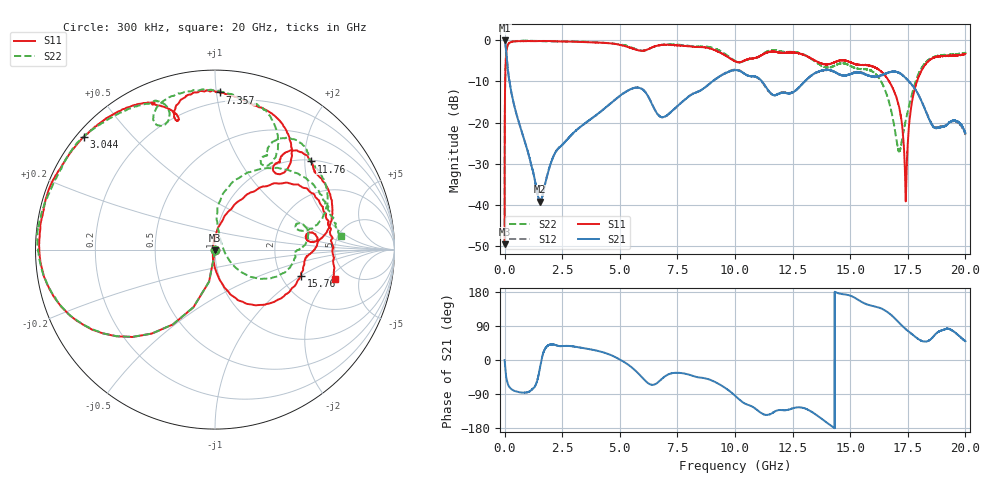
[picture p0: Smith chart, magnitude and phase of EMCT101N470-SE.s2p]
!EMCT101N470
!Johanson Technology Inc.
!www.johansontechnology.com
!Test Board Conditions:
!Substrate Type  RO4350B
!Substrate Thickness  10 mil
!Substrate Dk  3.66
!TL Type: GCPW
!TL Trace Width  22 mil
!TL Gap  14 mil
!PART MODE SINGLE ENDED (AKA BYPASS)
!DUT TOPOLOGY	SERIES-SHUNT
# MHz S  dB  R 50
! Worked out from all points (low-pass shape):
!   20001 points, 300 kHz to 20 GHz, reference 50 ohm
!   highest |S21| = -0.01 dB at 1.3 MHz (marker M1); lowest = -39.2 dB at 1.536 GHz (marker M2)
!   |S21| within 3 dB of the highest: start of sweep to 70.19 MHz
!   lowest |S11| = -49.6 dB at 300 kHz (marker M3), VSWR 1.01, Z = 50.2 - j0.292 ohm
!   |S11| at or under -10 dB: start of sweep to 23.99 MHz; 16.69105 GHz to 16.69105 GHz (0 Hz wide, 0 % of centre); 16.69 GHz to 17.9 GHz (1.208 GHz wide, 6.99 % of centre)
!   |S22| runs from -50.1 to 0.0 dB; largest |S21 - S12| = 0.0096
!   S11 on the Smith chart (normalised r, x): 300 kHz: 1.00, -0.01; 3.044 GHz: 0.02, +0.37; 7.357 GHz: 0.14, +1.02; 11.76 GHz: 1.03, +2.15; 15.76 GHz: 2.55, -1.00; 20 GHz: 3.79, -2.40
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0.3  -49.62 -61.7  -0.02 -0.4  -0.01 -0.3  -50.10 -65.6
1.3  -35.02 -87.8  -0.01 -1.1  -0.01 -1.1  -35.01 -87.5
101.298  -1.84 -146.2  -4.90 -55.2  -4.87 -55.2  -1.87 -146.0
157.298  -0.92 -157.6  -7.85 -65.9  -7.81 -66.0  -0.93 -157.1
1536.277  -0.14 164.4  -39.24 -20.0  -39.09 -19.3  -0.15 164.5
2172.267  -0.20 154.2  -27.64 40.2  -27.57 40.1  -0.27 155.7
3044.254  -0.33 139.3  -22.22 35.2  -22.23 34.9  -0.24 144.1
3334.25  -0.38 135.1  -20.84 32.2  -20.86 32.1  -0.27 140.6
5687.215  -2.22 105.6  -11.51 -28.5  -11.47 -28.2  -2.09 108.8
6667.2  -1.23 100.7  -18.16 -58.5  -18.11 -58.9  -1.21 110.3
7357.19  -1.15 88.1  -16.70 -34.2  -16.77 -34.1  -0.99 93.8
10000.15  -5.08 49.0  -7.22 -94.1  -7.12 -94.1  -4.99 57.4
11758.12  -2.77 42.5  -13.34 -135.0  -13.29 -134.1  -2.41 48.5
13334.1  -4.48 6.1  -8.48 -137.0  -8.48 -137.2  -4.59 14.0
15758.06  -6.01 -17.1  -8.50 146.3  -8.40 145.5  -7.06 -8.5
16667.05  -9.80 -62.9  -7.79 124.3  -7.82 125.3  -14.65 -40.6
17108.04  -15.88 -82.3  -7.88 99.3  -7.82 99.6  -26.90 12.3
17410.04  -39.09 -174.6  -9.16 81.6  -9.13 81.6  -19.45 78.9
17692.03  -14.65 74.7  -10.90 67.8  -10.98 68.1  -12.82 86.7
18129.03  -7.05 52.3  -15.25 49.8  -15.18 50.2  -6.45 65.3
18657.02  -4.17 31.2  -21.21 65.5  -21.12 65.2  -3.97 40.0
20000  -3.26 -14.1  -22.54 49.8  -22.83 51.0  -3.05 6.0
